| IBIS file was generated by Viper version: 2025.10.06
[IBIS Ver]   6.0
[Comment Char]   |_char
[File Name]   c15x_c05x_48qfn.ibs
[File Rev]   1.0
[Date]   Wed Oct 22 17:23:37 2025
[Source]   NXP Viper 2025.10.06
[Notes]
[Disclaimer] IMPORTANT NOTICE
  This information is provided on an AS IS basis and without warranty.
  IN NO EVENT SHALL NXP BE LIABLE FOR INCIDENTAL OR CONSEQUENTIAL
  DAMAGES ARISING FROM USE OF THIS INFORMATION. THIS DISCLAIMER OF
  WARRANTY EXTENDS TO THE USER OF THE INFORMATION, AND TO THEIR CUSTOMERS
  OR USERS OF PRODUCTS  AND IS IN LIEU OF ALL WARRANTIES WHETHER EXPRESS,
  IMPLIED, OR STATUTORY, INCLUDING IMPLIED WARRANTIES OF MERCHANTABILITY
  OR FITNESS FOR PARTICULAR PURPOSE.
  NXP does not represent or warrant that the information furnished
  hereunder is free of infringement of any third party patents,
  copyrights, trade secrets, or other intellectual property rights.
  NXP does not represent or warrant that the information is free of
  defect, or that it meets any particular standard, requirements or need
  of the user of the infomation or their customers.
  NXP reserves the right to change the information in this file
  without notice.
   http://www.nxp.com
[Copyright]   (C) Copyright NXP 2004 - 2025, All Rights Reserved.
|   C15x_C05x_48QFN
[Component]   C15x_C05x_48QFN
[Manufacturer]   NXP
[Package]
| variable   typ   min   max
R_pkg   0.31513   0.24777   0.41395
L_pkg   3.161e-09   2.281e-09   4.293e-09
C_pkg   2.002e-13   1.752e-13   2.522e-13
[Pin] signal_name   model_name   R_pin   L_pin   C_pin
1   P1_8   a_ip_io_3v_3p3v   0.33178   3.542e-09 2.193e-13
2   P1_9   a_ip_io_3v_3p3v   0.28874   3.196e-09 2.055e-13
3   P1_10   a_ip_io_3v_3p3v   0.26822   2.993e-09 1.955e-13
4   P1_11   a_ip_io_3v_3p3v   0.26167   2.812e-09 1.867e-13
5   P1_29   a_ip_io_3v_3p3v   0.25434   2.717e-09 1.772e-13
6   P1_30   a_ip_io_3v_3p3v   0.2529   2.560e-09 1.763e-13
7   P1_31   a_ip_io_3v_3p3v   0.27146   2.281e-09 1.991e-13
8   VDD_ANA   POWER   NA   NA   NA
9   VDD   POWER   NA   NA   NA
10   P2_0   a_ip_io_3v_3p3v   0.29228   2.889e-09 2.021e-13
11   P2_1   a_ip_io_3v_3p3v   0.31254   3.236e-09 2.257e-13
12   P2_2   a_ip_io_3v_3p3v   0.37272   3.961e-09 2.289e-13
13   P2_3   a_ip_io_3v_3p3v   0.3742   3.914e-09 2.180e-13
14   P2_6   a_ip_io_3v_3p3v   0.3396   3.458e-09 2.136e-13
15   P2_7   a_ip_io_3v_3p3v   0.32462   3.234e-09 1.978e-13
16   P2_12   a_ip_io_3v_3p3v   0.31758   2.977e-09 1.879e-13
17   P2_13   a_ip_io_3v_3p3v   0.3279   2.682e-09 1.957e-13
18   P2_16   a_ip_io_3v_3p3v   0.30436   2.928e-09 1.782e-13
19   P2_17   a_ip_io_3v_3p3v   0.30405   3.020e-09 1.802e-13
20   P2_20   a_ip_io_3v_3p3v   0.31259   3.137e-09 1.871e-13
21   P2_21   a_ip_io_3v_3p3v   0.32754   3.305e-09 1.937e-13
22   P2_28   a_ip_io_3v_3p3v   0.35089   3.551e-09 2.061e-13
23   P3_31   a_ip_io_3v_3p3v   0.37373   3.832e-09 2.306e-13
24   P3_30   a_ip_io_3v_3p3v   0.41395   4.293e-09 2.406e-13
25   P3_29   a_ip_io_3v_3p3v   0.40673   4.082e-09 2.253e-13
26   P3_28   a_ip_io_3v_3p3v   0.36228   3.352e-09 2.006e-13
27   P3_27   a_ip_io_3v_3p3v   0.36468   2.988e-09 2.107e-13
28   P3_14   a_ip_io_3v_3p3v   0.32764   3.109e-09 1.828e-13
29   P3_13   a_ip_io_3v_3p3v   0.31812   3.157e-09 1.779e-13
30   P3_12   a_ip_io_3v_3p3v   0.31342   3.165e-09 1.791e-13
31   P3_11   a_ip_io_3v_3p3v   0.31101   3.113e-09 1.776e-13
32   P3_10   a_ip_io_3v_3p3v   0.288   3.019e-09 1.794e-13
33   P3_9   a_ip_io_3v_3p3v   0.29682   3.097e-09 1.881e-13
34   P3_8   a_ip_io_3v_3p3v   0.30953   3.158e-09 2.009e-13
35   P3_1   a_ip_io_3v_3p3v   0.33124   3.225e-09 2.184e-13
36   P3_0   a_ip_io_3v_3p3v   0.3789   3.172e-09 2.522e-13
37   VDD   POWER   NA   NA   NA
38   P0_0   a_ip_io_3v_3p3v   0.32137   2.974e-09 2.113e-13
39   P0_1   a_ip_io_3v_3p3v   0.30341   3.081e-09 1.978e-13
40   P0_2   a_ip_io_3v_3p3v   0.29071   3.043e-09 1.889e-13
41   P0_3   a_ip_io_3v_3p3v   0.28103   2.965e-09 1.790e-13
42   P0_6   a_ip_io_3v_3p3v   0.27518   2.911e-09 1.752e-13
43   P0_16   a_ip_io_3v_3p3v   0.24777   2.818e-09 1.772e-13
44   P0_17   a_ip_io_3v_3p3v   0.25353   2.866e-09 1.817e-13
45   P1_0   a_ip_io_3v_3p3v   0.26505   2.976e-09 1.897e-13
46   P1_1   a_ip_io_3v_3p3v   0.28144   3.077e-09 2.007e-13
47   P1_2   a_ip_io_3v_3p3v   0.30927   3.198e-09 2.176e-13
48   P1_3   a_ip_io_3v_3p3v   0.36599   3.184e-09 2.505e-13
49   VSS   GND   NA   NA   NA
[Pin Mapping]   pulldown_ref   pullup_ref
1   VSS   VDD
2   VSS   VDD
3   VSS   VDD
4   VSS   VDD
5   VSS   VDD
6   VSS   VDD
7   VSS   VDD
8   NC   VDD_ANA
9   NC   VDD
10   VSS   VDD
11   VSS   VDD
12   VSS   VDD
13   VSS   VDD
14   VSS   VDD
15   VSS   VDD
16   VSS   VDD
17   VSS   VDD
18   VSS   VDD
19   VSS   VDD
20   VSS   VDD
21   VSS   VDD
22   VSS   VDD
23   VSS   VDD
24   VSS   VDD
25   VSS   VDD
26   VSS   VDD
27   VSS   VDD
28   VSS   VDD
29   VSS   VDD
30   VSS   VDD
31   VSS   VDD
32   VSS   VDD
33   VSS   VDD
34   VSS   VDD
35   VSS   VDD
36   VSS   VDD
37   NC   VDD
38   VSS   VDD
39   VSS   VDD
40   VSS   VDD
41   VSS   VDD
42   VSS   VDD
43   VSS   VDD
44   VSS   VDD
45   VSS   VDD
46   VSS   VDD
47   VSS   VDD
48   VSS   VDD
49   VSS   NC
|*   Model Selector   *
[Model Selector] a_ip_io_3v_3p3v
p_io_25mhz_ds0_sr0_3p3v_mio   dse=0 sre=0 25mhz
p_io_25mhz_ds0_sr1_3p3v_mio   dse=0 sre=1 25mhz
p_io_25mhz_ds1_sr0_3p3v_mio   dse=1 sre=0 25mhz
p_io_25mhz_ds1_sr1_3p3v_mio   dse=1 sre=1 25mhz
p_io_25mhz_r40_ds0_sr0_3p3v_mio   dse=0 sre=0 25mhz_r40
p_io_25mhz_r40_ds0_sr1_3p3v_mio   dse=0 sre=1 25mhz_r40
p_io_25mhz_r40_ds1_sr0_3p3v_mio   dse=1 sre=0 25mhz_r40
p_io_25mhz_r40_ds1_sr1_3p3v_mio   dse=1 sre=1 25mhz_r40
p_io_50mhz_ds0_sr0_3p3v_mio   dse=0 sre=0 50mhz
p_io_50mhz_ds0_sr1_3p3v_mio   dse=0 sre=1 50mhz
p_io_50mhz_ds1_sr0_3p3v_mio   dse=1 sre=0 50mhz
p_io_50mhz_ds1_sr1_3p3v_mio   dse=1 sre=1 50mhz
p_io_25mhz_cap_ds0_sr0_3p3v_mio   dse=0 sre=0 25mhz_cap
p_io_25mhz_cap_ds0_sr1_3p3v_mio   dse=0 sre=1 25mhz_cap
p_io_25mhz_cap_ds1_sr0_3p3v_mio   dse=1 sre=0 25mhz_cap
p_io_25mhz_cap_ds1_sr1_3p3v_mio   dse=1 sre=1 25mhz_cap
p_io_25mhz_2mux_ds0_sr0_3p3v_mio   dse=0 sre=0 25mhz_2mux
p_io_25mhz_2mux_ds0_sr1_3p3v_mio   dse=0 sre=1 25mhz_2mux
p_io_25mhz_2mux_ds1_sr0_3p3v_mio   dse=1 sre=0 25mhz_2mux
p_io_25mhz_2mux_ds1_sr1_3p3v_mio   dse=1 sre=1 25mhz_2mux
p_io_100mhz_ds0_sr0_3p3v_mio   dse=0 sre=0 100mhz
p_io_100mhz_ds0_sr1_3p3v_mio   dse=0 sre=1 100mhz
p_io_100mhz_ds1_sr0_3p3v_mio   dse=1 sre=0 100mhz
p_io_100mhz_ds1_sr1_3p3v_mio   dse=1 sre=1 100mhz
p_io_100mhz_weftd_ds0_sr0_3p3v_mio   dse=0 sre=0 100mhz
p_io_100mhz_weftd_ds0_sr1_3p3v_mio   dse=0 sre=1 100mhz
p_io_100mhz_weftd_ds1_sr0_3p3v_mio   dse=1 sre=0 100mhz
p_io_100mhz_weftd_ds1_sr1_3p3v_mio   dse=1 sre=1 100mhz
p_io_i2c_ds00_ds10_sr0_3p3v_mio   dse0=0 dse1=0 sre=0 i2c
p_io_i2c_ds00_ds10_sr1_3p3v_mio   dse0=0 dse1=0 sre=1 i2c
p_io_i2c_ds00_ds11_sr0_3p3v_mio   dse0=0 dse1=1 sre=0 i2c
p_io_i2c_ds00_ds11_sr1_3p3v_mio   dse0=0 dse1=1 sre=1 i2c
p_io_i2c_ds01_ds10_sr0_3p3v_mio   dse0=1 dse1=0 sre=0 i2c
p_io_i2c_ds01_ds10_sr1_3p3v_mio   dse0=1 dse1=0 sre=1 i2c
p_io_i2c_ds01_ds11_sr0_3p3v_mio   dse0=1 dse1=1 sre=0 i2c
p_io_i2c_ds01_ds11_sr1_3p3v_mio   dse0=1 dse1=1 sre=1 i2c
p_io_i2c_i2c1_3p3v_mio   ipp_i2c_lv=1 i2c
p_io_i2cfmp_ds00_ds10_sr0_3p3v_mio   dse0=0 dse1=0 sre=0 i2cfmp
p_io_i2cfmp_ds00_ds10_sr1_3p3v_mio   dse0=0 dse1=0 sre=1 i2cfmp
p_io_i2cfmp_ds00_ds11_sr0_3p3v_mio   dse0=0 dse1=1 sre=0 i2cfmp
p_io_i2cfmp_ds00_ds11_sr1_3p3v_mio   dse0=0 dse1=1 sre=1 i2cfmp
p_io_i2cfmp_ds01_ds10_sr0_3p3v_mio   dse0=1 dse1=0 sre=0 i2cfmp
p_io_i2cfmp_ds01_ds10_sr1_3p3v_mio   dse0=1 dse1=0 sre=1 i2cfmp
p_io_i2cfmp_ds01_ds11_sr0_3p3v_mio   dse0=1 dse1=1 sre=0 i2cfmp
p_io_i2cfmp_ds01_ds11_sr1_3p3v_mio   dse0=1 dse1=1 sre=1 i2cfmp
p_io_i2cfmp_i2c1_3p3v_mio   ipp_i2c_lv=1 i2cfmp
p_io_rst_3p3v_mio   rst
p_io_rst_rx1p8v_3p3v_mio   rst
p_io_aon_3p3v_mio   rst
| End [Component] C15x_C05x_48QFN
| Models and submodels in the file (49): p_io_100mhz_ds0_sr0_3p3v_mio (I/O), p_io_100mhz_ds0_sr1_3p3v_mio (I/O), p_io_100mhz_ds1_sr0_3p3v_mio (I/O), p_io_100mhz_ds1_sr1_3p3v_mio (I/O), p_io_100mhz_weftd_ds0_sr0_3p3v_mio (I/O), p_io_100mhz_weftd_ds0_sr1_3p3v_mio (I/O), p_io_100mhz_weftd_ds1_sr0_3p3v_mio (I/O), p_io_100mhz_weftd_ds1_sr1_3p3v_mio (I/O), p_io_25mhz_2mux_ds0_sr0_3p3v_mio (I/O), p_io_25mhz_2mux_ds0_sr1_3p3v_mio (I/O), p_io_25mhz_2mux_ds1_sr0_3p3v_mio (I/O), p_io_25mhz_2mux_ds1_sr1_3p3v_mio (I/O), p_io_25mhz_cap_ds0_sr0_3p3v_mio (I/O), p_io_25mhz_cap_ds0_sr1_3p3v_mio (I/O), p_io_25mhz_cap_ds1_sr0_3p3v_mio (I/O), p_io_25mhz_cap_ds1_sr1_3p3v_mio (I/O), p_io_25mhz_ds0_sr0_3p3v_mio (I/O), p_io_25mhz_ds0_sr1_3p3v_mio (I/O), p_io_25mhz_ds1_sr0_3p3v_mio (I/O), p_io_25mhz_ds1_sr1_3p3v_mio (I/O), p_io_25mhz_r40_ds0_sr0_3p3v_mio (I/O), p_io_25mhz_r40_ds0_sr1_3p3v_mio (I/O), p_io_25mhz_r40_ds1_sr0_3p3v_mio (I/O), p_io_25mhz_r40_ds1_sr1_3p3v_mio (I/O), p_io_50mhz_ds0_sr0_3p3v_mio (I/O), p_io_50mhz_ds0_sr1_3p3v_mio (I/O), p_io_50mhz_ds1_sr0_3p3v_mio (I/O), p_io_50mhz_ds1_sr1_3p3v_mio (I/O), p_io_aon_3p3v_mio (I/O), p_io_i2c_ds00_ds10_sr0_3p3v_mio (I/O), p_io_i2c_ds00_ds10_sr1_3p3v_mio (I/O), p_io_i2c_ds00_ds11_sr0_3p3v_mio (I/O), p_io_i2c_ds00_ds11_sr1_3p3v_mio (I/O), p_io_i2c_ds01_ds10_sr0_3p3v_mio (I/O), p_io_i2c_ds01_ds10_sr1_3p3v_mio (I/O), p_io_i2c_ds01_ds11_sr0_3p3v_mio (I/O), p_io_i2c_ds01_ds11_sr1_3p3v_mio (I/O), p_io_i2c_i2c1_3p3v_mio (I/O), p_io_i2cfmp_ds00_ds10_sr0_3p3v_mio (I/O), p_io_i2cfmp_ds00_ds10_sr1_3p3v_mio (I/O), p_io_i2cfmp_ds00_ds11_sr0_3p3v_mio (I/O), p_io_i2cfmp_ds00_ds11_sr1_3p3v_mio (I/O), p_io_i2cfmp_ds01_ds10_sr0_3p3v_mio (I/O), p_io_i2cfmp_ds01_ds10_sr1_3p3v_mio (I/O), p_io_i2cfmp_ds01_ds11_sr0_3p3v_mio (I/O), p_io_i2cfmp_ds01_ds11_sr1_3p3v_mio (I/O), p_io_i2cfmp_i2c1_3p3v_mio (I/O), p_io_rst_3p3v_mio (I/O), p_io_rst_rx1p8v_3p3v_mio (I/O)
